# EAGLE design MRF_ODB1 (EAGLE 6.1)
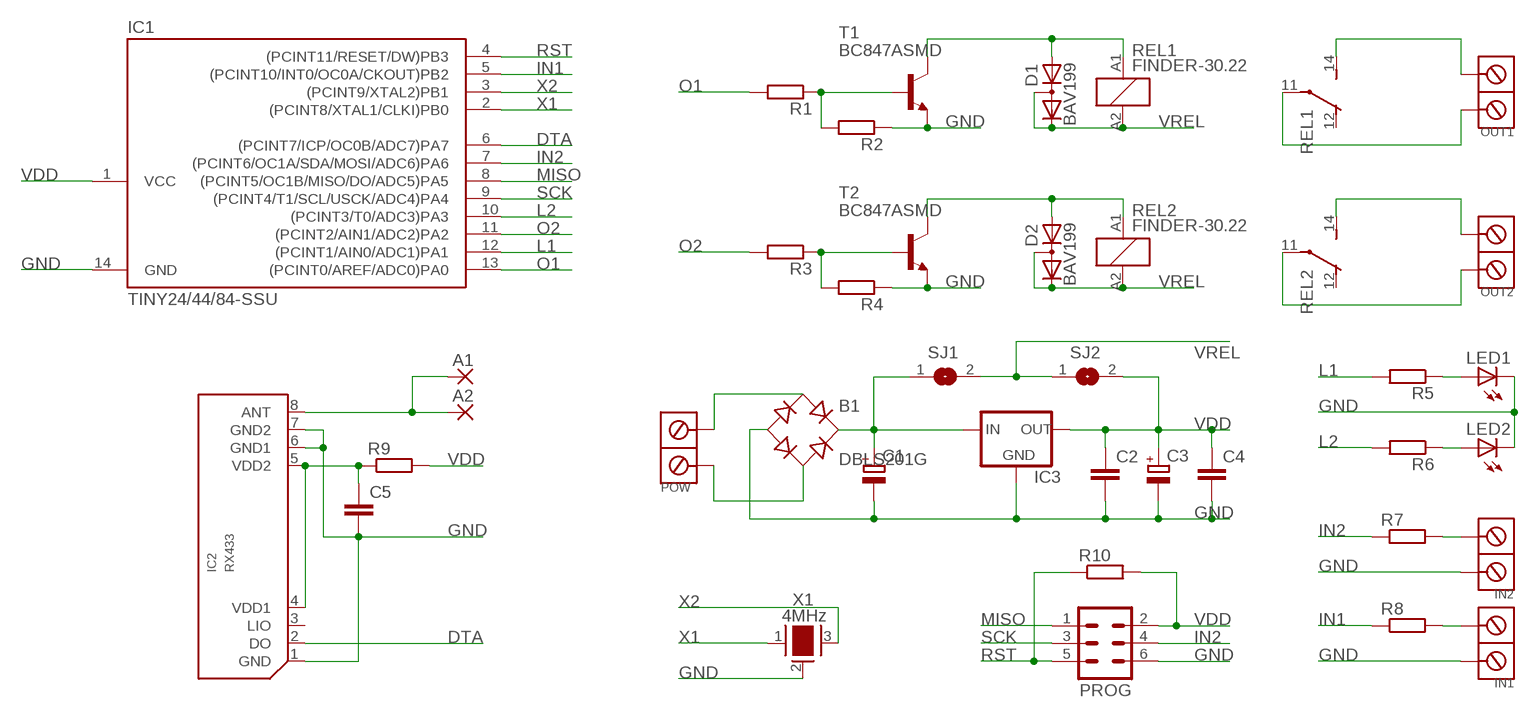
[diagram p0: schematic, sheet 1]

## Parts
A1  2,54/1,0  [2,54/1,0]
A2  2,54/1,0  [2,54/1,0]
B1  DBLS201G  [DBS]
C1  CPOL-EUE2.5-7  [E2,5-7]
C2  C-EUC0805K  [C0805K]
C3  CPOL-EUE2.5-7  [E2,5-7]
C4  C-EUC0805K  [C0805K]
C5  C-EUC0805K  [C0805K]
D1  BAV199  [SOT23]
D2  BAV199  [SOT23]
IC1  TINY24/44/84-SSU  [SOIC14]
IC2  RX433  [RX433]
IC3  78XXL  [78XXL]
IN1  ARK2ARK2/500  [ARK2/500]
IN2  ARK2ARK2/500  [ARK2/500]
LED1  LED3MM  [LED3MM]
LED2  LED3MM  [LED3MM]
OUT1  ARK2  [ARK2/750]
OUT2  ARK2  [ARK2/750]
POW  ARK2ARK2/500  [ARK2/500]
PROG  MA03-2  [MA03-2]
R1  R-EU_R0805  [R0805]
R2  R-EU_R0805  [R0805]
R3  R-EU_R0805  [R0805]
R4  R-EU_R0805  [R0805]
R5  R-EU_R0805  [R0805]
R6  R-EU_R0805  [R0805]
R7  R-EU_R0805  [R0805]
R8  R-EU_R0805  [R0805]
R9  R-EU_R0805  [R0805]
R10  R-EU_R0805  [R0805]
REL1  FINDER-30.22  [FINDER-30.22]
REL2  FINDER-30.22  [FINDER-30.22]
SJ1  SJ  [SJ]
SJ2  SJ  [SJ]
T1  BC847ASMD  [SOT23]
T2  BC847ASMD  [SOT23]
X1  4MHz  Q4M_SMD  [Q4M_SMD]

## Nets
DTA: IC1.6((PCINT7/ICP/OC0B/ADC7)PA7) IC2.2(DO)
GND: B1.- C1.- C2.2 C3.- C4.2 C5.2 IC1.14(GND) IC2.1(GND) IC2.6(GND1) IC2.7(GND2) IC3.GND IN1.1 IN2.1 LED1.K(C) LED2.K(C) PROG.6 R2.1 R4.1 T1.2(E) T2.2(E) X1.2
IN1: IC1.5((PCINT10/INT0/OC0A/CKOUT)PB2) R8.1
IN2: IC1.7((PCINT6/OC1A/SDA/MOSI/ADC6)PA6) PROG.4 R7.1
L1: IC1.12((PCINT1/AIN0/ADC1)PA1) R5.2
L2: IC1.10((PCINT3/T0/ADC3)PA3) R6.2
MISO: IC1.8((PCINT5/OC1B/MISO/DO/ADC5)PA5) PROG.1
N$1: R3.1 R4.2 T2.1(B)
N$2: D2.1(A) REL2.A1 T2.3(C)
N$3: C5.1 IC2.4(VDD1) IC2.5(VDD2) R9.1
N$4: B1.AC1 POW.2
N$5: B1.AC2 POW.1
N$6: LED1.A R5.1
N$7: LED2.A R6.1
N$8: R1.1 R2.2 T1.1(B)
N$9: IN1.2 R8.2
N$10: IN2.2 R7.2
N$11: D1.1(A) REL1.A1 T1.3(C)
N$12: OUT1.2 REL1.14(-1:S)
N$13: OUT1.1 REL1.11(-1:P)
N$14: OUT2.2 REL2.14(-1:S)
N$15: A1.1(P) A2.1(P) IC2.8(ANT)
N$16: OUT2.1 REL2.11(-1:P)
N$23: B1.+ C1.+ IC3.IN SJ1.1
O1: IC1.13((PCINT0/AREF/ADC0)PA0) R1.2
O2: IC1.11((PCINT2/AIN1/ADC2)PA2) R3.2
RST: IC1.4((PCINT11/RESET/DW)PB3) PROG.5 R10.1
SCK: IC1.9((PCINT4/T1/SCL/USCK/ADC4)PA4) PROG.3
VDD: C2.1 C3.+ C4.1 IC1.1(VCC) IC3.OUT PROG.2 R9.2 R10.2 SJ2.2
VREL: D1.2(C) D1.3(AC) D2.2(C) D2.3(AC) REL1.A2 REL2.A2 SJ1.2 SJ2.1
X1: IC1.2((PCINT8/XTAL1/CLKI)PB0) X1.1
X2: IC1.3((PCINT9/XTAL2)PB1) X1.3
Unconnected: IC2.3(LIO) REL1.12(-1:O) REL1.21(-2:P) REL1.22(-2:O) REL1.24(-2:S) REL2.12(-1:O) REL2.21(-2:P) REL2.22(-2:O) REL2.24(-2:S)

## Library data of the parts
A1 A2 = wirepad:2,54/1,0: THROUGH-HOLE PAD
B1 = rectifier:DB?*G: Single Phase 1.0 AMP Glass Passivated Bridge Rectifier Taiwan Semiconductor Co.,Ltd. - TSC Source: http://www.taiwansemi.com/TSCbig5/ezcatfiles/cust/img/img/db101g.pdf http://www.ts.com.tw/db/pictures/modules/PDT/PDT060207001/DBLS201G.pdf
C1 C3 = rcl:CPOL-EU: POLARIZED CAPACITOR, European symbol
C2 C4 C5 = rcl:C-EU: CAPACITOR, European symbol
D1 D2 = diode:BAV199: DIODE low-leakage double diode
IC1 = avr-7:TINY24/44/84
IC2 = RF:RX433
IC3 = v-reg:78XXL: VOLTAGE REGULATOR
IN1 IN2 OUT1 OUT2 POW = dimmer:ARK2
LED1 LED2 = led:LED: LED
PROG = con-lstb:MA03-2: PIN HEADER; OC_FARNELL: unknown; OC_NEWARK: unknown
R1-R10 = rcl:R-EU_: RESISTOR, European symbol
REL1 REL2 = relay:FINDER-30.22: SUBMINIATURE DIL-RELAIS FINDER 30.22.9.024.0000 Kontakt max. AC - 125V Distributor: Farnell Bestell Nr.: 1217371 Source: http://www.farnell.com/datasheets/87634.pdf; OC_FARNELL: unknown; OC_NEWARK: unknown
SJ1 SJ2 = jumper:SJ: SMD solder JUMPER
T1 T2 = transistor-npn:BC847*: NPN Transistor
X1 = DS:Q4M_SMD

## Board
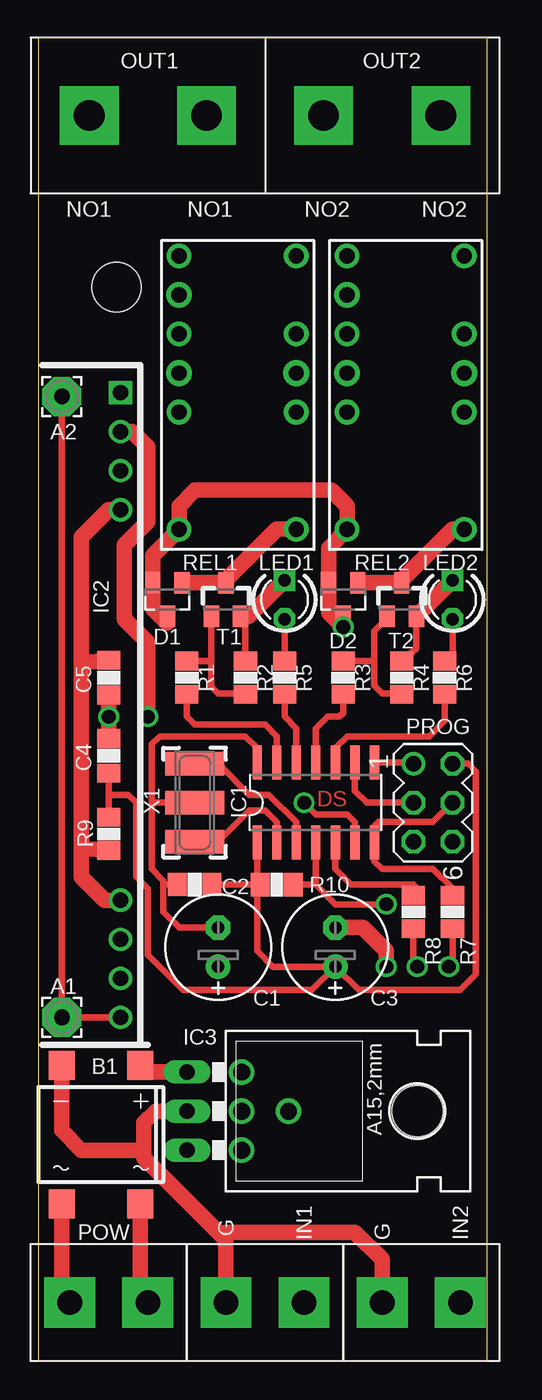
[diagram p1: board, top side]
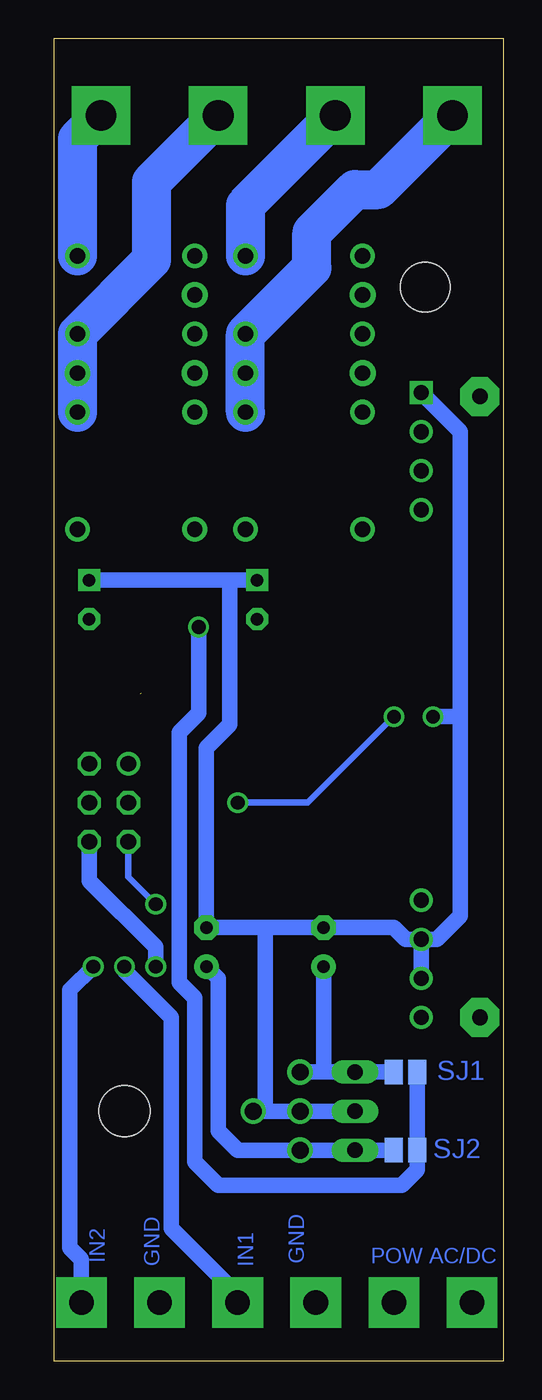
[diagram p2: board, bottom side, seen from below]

Size 29.19 x 86.03 mm. Coordinates in mm from the lower left corner, seen from the top.
Outline: 0,0 29.19,0 29.19,86.03 0,86.03 0,0
Copper layers (1*16): Top 0.035mm / dielectric 1.5mm / Bottom 0.035mm
Design rules: minimum track width 10mil, minimum drill 24mil, track to track 8mil, track to pad 8mil, pad to pad 8mil, via to via 8mil, smd to smd 8mil, copper to edge 40mil, drill to drill 8mil, minimum pad ring 10mil, minimum via ring 8mil, stop-mask expansion 4mil, vias tented up to drill 0mil, thermal gap 10mil
Holes 3.2 mm at 5.08,69.85

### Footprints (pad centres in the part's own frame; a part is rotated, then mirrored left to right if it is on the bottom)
2,54/1,0 = drill 1.016 pad 2.54 octagon: 1 0,0
DBS = smd 1.7 x 1.9: + -2.55,-4.5; - 2.55,-4.5; AC1 -2.55,4.5; AC2 2.55,4.5
E2,5-7 = drill 0.813 pad 1.6: + -1.27,0 | drill 0.813 pad 1.6 octagon: - 1.27,0
C0805K = smd 1.219 x 1.499: 1 -1.127,0; 2 1.127,0
SOT23 = smd 1 x 1.4: 1 -0.95,-1.1; 2 0.95,-1.1; 3 0,1.1
SOIC14 = smd 0.61 x 2.21: 1 -3.81,-2.603; 2 -2.54,-2.603; 3 -1.27,-2.603; 4 0,-2.603; 5 1.27,-2.603; 6 2.54,-2.603; 7 3.81,-2.603; 8 3.81,2.603; 9 2.54,2.603; 10 1.27,2.603; 11 0,2.603; 12 -1.27,2.603; 13 -2.54,2.603; 14 -3.81,2.603
RX433 = drill 1 square: 1 -20.32,0 | drill 1: 2 -17.78,0; 3 -15.24,0; 4 -12.7,0; 5 12.7,0; 6 15.24,0; 7 17.78,0; 8 20.32,0
78XXL = drill 1.016 long: GND 0,-3.81; IN -2.54,-3.81; OUT 2.54,-3.81 | hole 3.302: 0,11.176
ARK2/500 = drill 1.6 pad 3.302 square: 1 -2.54,0; 2 2.54,0
LED3MM = drill 0.813 pad 1.422 octagon: A -1.27,0 | drill 0.813 pad 1.422 square: K 1.27,0
ARK2/750 = drill 2 pad 3.81 square: 1 -3.81,0; 2 3.81,0
MA03-2 = drill 1.016: 1 -2.54,-1.27 | drill 1.016 octagon: 2 -2.54,1.27; 3 0,-1.27; 4 0,1.27; 5 2.54,-1.27; 6 2.54,1.27
R0805 = smd 1.219 x 1.5: 1 -1.077,0; 2 1.077,0
FINDER-30.22 = drill 1 pad 1.6: 11 -1.27,-3.81; 12 3.81,-3.81; 14 8.89,-3.81; 21 -1.27,3.81; 22 3.81,3.81; 24 8.89,3.81; A1 -8.89,-3.81; A2 -8.89,3.81
SJ = smd 1.168 x 1.6: 1 -0.762,0; 2 0.762,0
Q4M_SMD = smd 1.524 x 3.81: 1 -2.54,0; 2 0,0; 3 2.54,0

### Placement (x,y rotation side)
A1  1.52,22.35 0 top
A2  1.52,62.74 0 top
B1  4.06,14.73 180 top
C1  11.68,26.92 90 top
C2  10.16,30.99 180 top
C3  19.3,26.92 90 top
C4  4.57,39.37 90 top
C5  4.57,44.45 270 top
D1  8.38,49.53 180 top
D2  19.81,49.53 180 top
IC1  18.03,36.32 0 top
IC2  5.33,42.67 270 top
IC3  13.46,16.26 270 top
IN1  14.73,3.81 0 top
IN2  24.89,3.81 0 top
LED1  16,49.53 90 top
LED2  26.92,49.53 90 top
OUT1  7.11,81.03 0 top
OUT2  22.35,81.03 0 top
POW  4.57,3.81 0 top
PROG  25.65,36.32 270 top
R1  9.65,44.45 270 top
R2  13.46,44.45 270 top
R3  19.81,44.45 270 top
R4  23.62,44.45 270 top
R5  16,44.45 270 top
R6  26.42,44.45 270 top
R7  26.92,29.21 270 top
R8  24.38,29.21 270 top
R9  4.57,34.29 90 top
R10  15.49,30.99 180 top
REL1  12.95,62.99 90 top
REL2  23.88,62.99 90 top
SJ1  6.35,18.8 0 bottom
SJ2  6.35,13.72 180 bottom
T1  12.19,49.53 0 top
T2  23.62,49.53 0 top
X1  10.16,36.32 90 top

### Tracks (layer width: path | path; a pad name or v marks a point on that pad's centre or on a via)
DTA  (via drill 0.9)
  Top 0.406: IC1.6 20.57,35.05 20.07,35.56 18.03,35.56 v17.27,36.32
  Top 1.016: v7.11,41.91 7.11,46.74 5.59,48.26 5.59,53.09 7.11,54.61 7.11,59.44 6.1,60.45 IC2.2
  Bottom 0.406: v17.27,36.32 12.7,36.32 v7.11,41.91
GND  (via drill 0.9, 1.1)
  Top 0.406: IC1.14 14.22,39.88 13.46,40.64 7.87,40.64 7.37,40.13 7.37,36.32 | 7.37,36.32 7.37,32 8.13,31.24 8.13,30.99 | 8.13,30.99 8.13,29.21 9.14,28.19 C1.- | X1.2 7.37,36.32 | C2.2 8.13,30.99 | T2.2 24.57,46.35 R4.1 | R2.1 13.46,48.11 T1.2
  Top 1.016: B1.- 1.51,15 2.79,13.72 6.86,13.72 | 6.86,13.72 6.86,15.49 7.62,16.26 IC3.GND | IN1.1 12.19,7.87 | 12.19,8.13 12.19,8.38 | 12.19,8.13 12.19,7.87 | 12.19,7.87 6.86,13.21 6.86,13.72 | IN2.1 22.35,6.6 20.57,8.38 12.45,8.38 12.19,8.13 | C4.2 v4.57,41.91 C5.2 | T2.2 24.55,48.43 LED2.K | T1.2 13.63,48.43 LED1.K | v22.61,25.65 22.61,26.67 21.08,28.19 C3.-
  Bottom 1.016: 15.49,28.19 15.49,16.51 15.24,16.26 | 15.49,28.19 C3.- 19.3,39.88 17.78,41.4 17.78,50.8 | 15.49,28.19 C1.- 7.11,28.19 6.35,27.43 IC2.6 | IC2.7 IC2.6 | IC2.1 2.79,60.45 2.79,41.91 | 2.79,41.91 2.79,28.96 4.32,27.43 IC2.6 | v4.57,41.91 2.79,41.91 | LED1.K 17.78,50.8 | 17.78,50.8 LED2.K | PROG.6 26.92,31.24 22.61,26.92 v22.61,25.65 | IC3.GND v13.21,16.26 15.24,16.26 | 15.24,16.26 v16.26,16.26
IN1
  Top 0.406: IC1.5 19.3,32 20.32,30.99 24.38,30.99 24.89,30.48 R8.1
IN2
  Top 0.406: PROG.4 25.65,35.05 22.1,35.05 21.84,34.8 IC1.7 21.84,32.51 22.35,32 25.65,32 26.92,30.73 R7.1
L1
  Top 0.406: IC1.12 16.76,41.15 16,41.91 R5.2
L2
  Top 0.406: R6.2 26.42,41.66 25.4,40.64 20.07,40.64 19.3,39.88 IC1.10
MISO
  Top 0.406: IC1.8 24.57,38.93 PROG.1
N$1  (1 unrouted)
  Top 0.406: T2.1 22.67,48.33 21.84,47.5 21.84,45.53 | 21.84,45.53 21.84,43.94 22.35,43.43 23.56,43.43 | R3.1 21.84,45.53
N$2
  Top 1.016: D2.1 T2.3 23.62,50.8 26.92,54.1 REL2.A1
N$3
  Top 1.016: R9.1 2.86,33.34 2.79,33.27 | 2.79,33.27 2.79,31.5 4.32,29.97 IC2.5 | IC2.4 4.57,55.37 2.79,53.59 2.79,45.72 | 2.79,45.72 2.79,33.27 | C5.1 2.81,45.45 2.79,45.72
N$4
  Top 1.016: B1.AC1 6.61,4.31 POW.2
N$5
  Top 1.016: B1.AC2 1.51,4.33 POW.1
N$6
  Top 0.406: LED1.A R5.1
N$7
  Top 0.406: LED2.A 26.92,45.91 R6.1
N$8
  Top 0.406: T1.1 11.24,45.53 | R2.2 13.4,43.43 11.68,43.43 11.24,43.88 11.24,45.47 11.24,45.53 | R1.1 11.24,45.53
N$9  (via drill 0.9)
  Top 0.406: R8.2 24.38,25.91 v24.64,25.65
  Bottom 1.016: IN1.2 17.27,4.32 21.59,8.64 21.59,22.35 24.64,25.4 v24.64,25.65
N$10  (via drill 0.9)
  Top 0.406: R7.2 26.92,25.91 v26.67,25.65
  Bottom 1.016: v26.67,25.65 28.19,24.13 28.19,7.37 27.43,6.6 IN2.2
N$11
  Top 1.016: D1.1 T1.3 12.19,50.8 15.49,54.1 REL1.A1
N$12
  Bottom 2.54: OUT1.2 16.76,75.18 REL1.14
N$13
  Bottom 2.54: REL1.11 16.76,66.8 12.45,71.12 12.45,73.41 9.65,76.2 8.13,76.2 OUT1.1
N$14
  Bottom 2.54: REL2.14 27.69,79.5 OUT2.2
N$15
  Top 0.406: IC2.8 A1.1 A2.1
N$16
  Bottom 2.54: REL2.11 27.69,66.8 22.86,71.63 22.86,76.71 OUT2.1
N$17  (via drill 1 pad 1.68)
  other vias: 27.69,64.26
N$18  (via drill 1 pad 1.68)
  other vias: 16.76,64.26
N$19  (via drill 1 pad 1.68)
  other vias: 20.07,69.34
N$20  (via drill 1 pad 1.68)
  other vias: 9.14,69.34
N$21  (via drill 1 pad 1.68)
  other vias: 9.14,64.26
N$22  (via drill 1 pad 1.68)
  other vias: 20.07,64.26
N$23  (via drill 1.1)
  Top 1.016: IC3.IN 6.6,18.8 6.35,19.24 B1.+
  Bottom 1.016: C1.+ 11.68,18.8 | 11.68,18.8 IC3.IN SJ1.1 | 11.68,18.8 v13.21,18.8
O1
  Top 0.406: IC1.13 15.49,40.64 14.73,41.4 10.16,41.4 9.65,41.91 R1.2
O2
  Top 0.406: IC1.11 18.03,41.15 18.8,41.91 19.56,41.91 19.81,42.16 R3.2
RST  (via drill 0.9)
  Top 0.406: IC1.4 18.03,30.99 | R10.1 18.03,30.99 | 18.03,30.99 19.3,29.72 v22.61,29.72
  Bottom 0.406: PROG.5 24.38,31.5 v22.61,29.72
SCK
  Top 0.406: PROG.3 21.34,36.32 20.57,37.08 IC1.9
VDD  (via drill 1.1)
  Top 0.406: C3.+ 17.78,24.13 9.4,24.13 7.11,26.42 7.11,30.73 6.35,31.5 6.35,36.32 5.84,36.83 4.57,36.83 | 4.57,36.83 C4.1 | R9.2 4.57,36.83 | IC1.1 14.22,30.99 | 14.22,30.99 14.22,26.67 15.24,25.65 C3.+ | C2.1 14.22,30.99 | R10.2 14.22,30.99 | PROG.2 27.94,38.86 28.45,38.35 28.45,25.15 27.43,24.13 20.83,24.13 C3.+
  Bottom 1.016: C3.+ 18.54,24.89 18.54,14.99 17.27,13.72 v13.21,13.72 IC3.OUT SJ2.2
VREL  (via drill 0.9)
  Top 1.016: D1.3 8.38,48.01 7.43,48.96 D1.2 7.43,52.39 REL1.A2 9.14,55.63 10.16,56.64 19.05,56.64 20.07,55.63 REL2.A2 18.86,52.9 D2.2 18.86,48.7 v19.81,47.75 D2.3
  Bottom 1.016: v19.81,47.75 19.81,42.16 21.08,40.89 21.08,24.64 20.07,23.62 20.07,12.95 18.54,11.43 6.6,11.43 5.59,12.45 SJ2.1 SJ1.2
X1
  Top 0.406: IC1.2 15.49,35.05 14.73,35.81 13.72,35.81 11.68,33.78 X1.1
X2
  Top 0.406: IC1.3 16.76,35.05 14.99,36.83 13.72,36.83 11.68,38.86 X1.3

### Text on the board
Top: DS
Bottom: SJ1 | SJ2 | GND | IN1 | IN2 | POW AC/DC | GND
tPlace: NO1 | NO1 | NO2 | NO2
tNames: G | G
